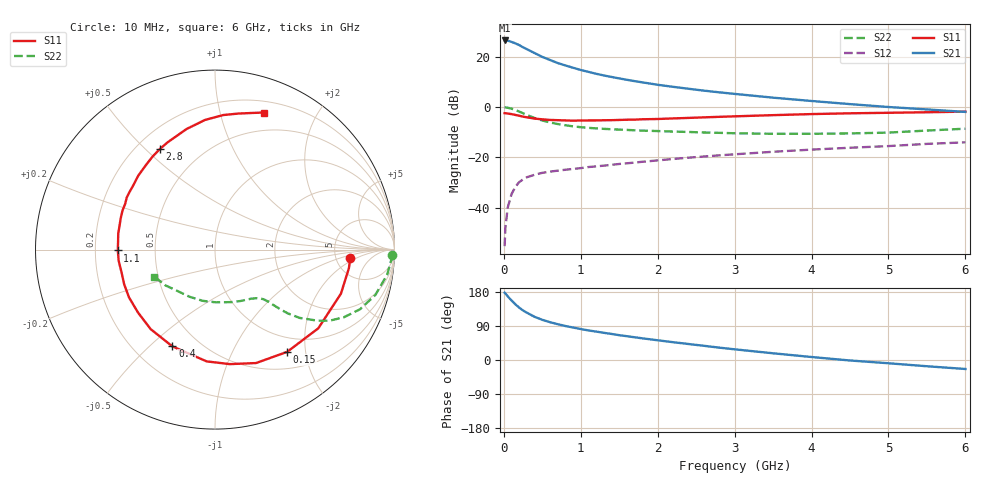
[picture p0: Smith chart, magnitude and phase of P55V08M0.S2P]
! SIEMENS Small Signal Semiconductors
! BFP183
! Si NPN RF Bipolar Junction Transistor in SOT143
! VCE = 5 V  IC = 8 mA
! Common Emitter S-Parameters:  March  1996
# GHz  S  MA  R  50
!  f  S11  S21  S12  S22
! GHz  MAG  ANG  MAG  ANG  MAG  ANG  MAG  ANG
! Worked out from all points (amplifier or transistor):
!   36 points, 10 MHz to 6 GHz, reference 50 ohm
!   highest |S21| = 26.5 dB at 10 MHz (marker M1)
!   |S21| within 3 dB of that: start of sweep to 267.8 MHz
!   unconditionally stable (mu >= 1): 1.319 GHz to 5.642 GHz
!   at 250 MHz: K = 0.28, MSG = 26.3 dB, |S12| = -28.8 dB
!   at 1.4 GHz: K = 1.03, MAG = 16.5 dB, |S12| = -23.0 dB
!   at 6 GHz: K = 0.95, MSG = 6.1 dB, |S12| = -14.0 dB
!   lowest NFmin = 1.30 dB at 450 MHz
!   S11 on the Smith chart (normalised r, x): 10 MHz: 6.82, -1.55; 150 MHz: 0.75, -1.67; 400 MHz: 0.36, -0.59; 1.1 GHz: 0.30, -0.00; 2.8 GHz: 0.29, +0.55; 6 GHz: 0.31, +1.37
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0.01  0.7555 -3.7  21.17 177.5  0.0017 83.2  0.988 -1.6
0.02  0.7532 -7.9  21.15 175.6  0.0039 79.8  0.9841 -3.3
0.05  0.7433 -19.3  20.98 168.1  0.0099 82.4  0.9697 -8.2
0.1  0.7236 -37.3  19.82 157.1  0.0185 71.6  0.9285 -15.8
0.15  0.6972 -54.8  18.54 146.9  0.0258 64.3  0.8735 -22.4
0.2  0.6722 -70.1  17.11 138.1  0.0321 58.0  0.8108 -27.7
0.25  0.6434 -82.6  15.48 130.7  0.0363 53.2  0.7516 -31.8
0.3  0.6245 -94.3  14.15 124.7  0.0401 49.8  0.6961 -34.7
0.4  0.5892 -113.8  11.84 113.9  0.0449 44.8  0.6061 -38.9
0.5  0.5698 -129.0  9.967 106.0  0.049 41.4  0.5399 -41.2
0.6  0.5541 -140.7  8.653 99.8  0.0518 39.5  0.4942 -42.4
0.7  0.5482 -150.9  7.524 94.5  0.0541 39.1  0.4593 -43.2
0.9  0.5359 -166.3  6.058 85.7  0.0586 38.1  0.4127 -44.4
1.1  0.5416 -179.5  5.014 78.0  0.0639 38.4  0.3852 -45.8
1.3  0.5465 170.6  4.254 71.7  0.0682 38.5  0.3679 -47.6
1.6  0.5594 157.1  3.489 62.8  0.0759 39.3  0.3505 -50.8
2.2  0.5937 136.1  2.528 47.0  0.0925 39.2  0.3252 -60.2
2.8  0.6387 118.9  1.964 32.6  0.1093 36.9  0.3067 -72.4
3.5  0.6902 103.3  1.538 17.7  0.1288 33.7  0.2936 -89.3
4.5  0.7511 86.5  1.144 -1.3  0.1549 27.3  0.2986 -118.4
5.5  0.788 75.0  0.897 -16.5  0.1848 21.2  0.3405 -144.2
6  0.811 70.3  0.8 -23.7  0.1985 17.0  0.3709 -156.0
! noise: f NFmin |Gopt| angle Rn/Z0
0.45  1.3  0.17  43  0.21
0.9  1.35  0.21  115  0.2
1.8  2.05  0.33  -177  0.14
